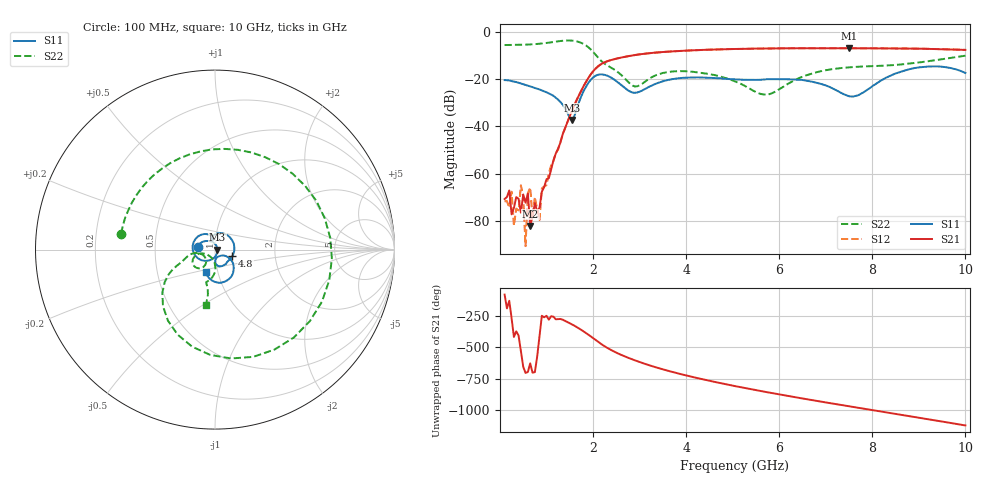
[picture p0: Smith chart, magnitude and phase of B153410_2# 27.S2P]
!  2-Port S-parameters saved by WinCal
! VAR MeasName=S-Parameters (CALIBRATED_DATA) read from VNA (N5245A)
! VAR MeasDate=2016-12-23 10:00:44
! VAR NAME=B153410_2# 27
! VAR FILENAME=B153410_2# 27.S2P
! VAR DATE=2016-12-23 10:00:44
! VAR PHYS_PORTS=1,2
# Hz S DB R 50
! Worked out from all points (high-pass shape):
!   199 points, 100 MHz to 10 GHz, reference 50 ohm
!   highest |S21| = -6.86 dB at 7.5 GHz (marker M1); lowest = -82.2 dB at 650 MHz (marker M2)
!   |S21| within 3 dB of the highest: 2.87 GHz to end of sweep
!   lowest |S11| = -37.3 dB at 1.55 GHz (marker M3), VSWR 1.03, Z = 51.4 + j0.0169 ohm
!   |S11| at or under -10 dB: start of sweep to end of sweep
!   |S22| runs from -26.5 to -3.6 dB; largest |S21 - S12| = 0.0035
!   S11 on the Smith chart (normalised r, x): 100 MHz: 0.83, +0.02; 4.8 GHz: 1.21, -0.09; 10 GHz: 0.87, -0.22
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1e8  -20.38 172.7  -70.79 -79.3  -71.76 -141.4  -5.52 170.3
2e8  -20.55 165.1  -67.13 -129.1  -74.44 63.4  -5.50 160.4
2.5e8  -20.81 161.1  -77.27 91.7  -67.69 -10.7  -5.51 155.3
3e8  -21.02 157.8  -74.56 -57.1  -82.00 -97.5  -5.48 150.3
4.5e8  -21.79 148.1  -76.60 -168.8  -64.97 -15.9  -5.42 134.3
5.5e8  -22.40 142.6  -72.33 15.7  -90.77 -163.0  -5.36 123.1
6.5e8  -23.02 137.6  -82.23 92.3  -65.97 -1.0  -5.26 111.1
7e8  -23.36 135.3  -78.15 17.6  -78.82 154.0  -5.21 104.9
7.5e8  -23.73 132.2  -72.56 22.6  -69.98 88.1  -5.14 98.3
8.5e8  -24.34 127.5  -74.45 -50.2  -79.63 -4.7  -4.98 84.4
9e8  -24.73 124.6  -67.70 111.2  -66.30 90.3  -4.88 77.1
1.55e9  -37.26 0.7  -33.22 42.2  -33.16 42.2  -3.64 -48.2
1.75e9  -27.07 -95.0  -24.72 -1.5  -24.74 -1.6  -4.62 -92.6
2.15e9  -17.96 170.7  -13.92 -107.4  -13.90 -107.3  -11.74 -155.0
2.85e9  -25.68 104.0  -9.92 123.0  -9.91 123.1  -22.70 -155.4
3.4e9  -21.54 91.6  -8.63 55.1  -8.63 55.1  -17.95 -125.8
4.8e9  -19.73 -20.3  -7.31 -70.2  -7.31 -70.0  -19.21 -163.8
5.05e9  -20.05 -31.5  -7.18 -89.1  -7.19 -88.9  -20.90 -165.6
6.7e9  -21.04 -82.0  -6.86 159.5  -6.88 159.6  -17.61 -91.4
7.5e9  -27.22 -71.5  -6.86 110.1  -6.89 110.1  -14.97 -102.5
8.35e9  -18.86 -34.6  -6.94 58.5  -6.93 58.8  -14.12 -104.0
1e10  -17.35 -112.8  -7.57 -42.9  -7.57 -42.7  -10.02 -99.4
